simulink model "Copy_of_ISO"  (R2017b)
settings: Solver=FixedStepDiscrete  StartTime=0.0  StopTime=10.0  FixedStep=0.01  RelTol=1e-3  EnableMultiTasking=on
undefined symbols (not defined in the file): ASWTYPE_FALSE, ASWTYPE_TRUE, CcISO_CTCOnlineDelayTime_ms, CcISO_FirLvlDebTime_ms, CcISO_FirLvlResChrg_kohm, CcISO_FirLvlResNotChrg_kohm, CcISO_InitDiagDebMaxTi_ms, CcISO_InitDiagDebTi_ms, CcISO_IsoDefaultValue_kohm, CcISO_IsoMeasDelayTime_ms, CcISO_ISONegVoltDebTime_ms, CcISO_ISONegVoltFliterDiff_V, CcISO_ISOPackVoltMax_V, CcISO_ISOPackVoltMin_V, CcISO_ISOResCnfFltCnt_NUMB, CcISO_ISOResCnfFltVal_kohm, CcISO_ISOResCnfWarnCnt_NUMB, CcISO_ISOResCnfWarnVal_kohm, CcISO_ISOResNvmMin_kohm, CcISO_IsoResVldVal_NUMB, CcISO_ISOSlopeDelayTime_ms, CcISO_ISOSlopeFilterVal_NUMB, CcISO_NegStMeasFiltTi_ms, CcISO_NegVoltHighRat_pct, CcISO_NegVoltLowRat_pct, CcISO_NorLvlResChrg_kohm, CcISO_NorLvlResNotChrg_kohm, CcISO_PosStMeasFiltTi_ms, CcISO_SedLvlDebTime_ms, CcISO_SedLvlResChrg_kohm, CcISO_SedLvlResNotChrg_kohm, Enum_CTCCtrCtlConnMode, Enum_CTCCtrCtlState, Enum_ISOHVIsoFltLevel, Enum_ISOHVIsoMeasState, Enum_LDPCC2St, Enum_MSMBMUState, ISO_CONST0_NUMB, ISO_CONST1000_NUMB, ISO_CONST1_NUMB, ISO_RESRB1_OHM, ISO_RESRB2_OHM, ISO_RESRS1_OHM, ISO_RESRS2_OHM, ISO_RUNTIME_MS
libraries: AIWAYS_Powertrain_BMS_lib x48
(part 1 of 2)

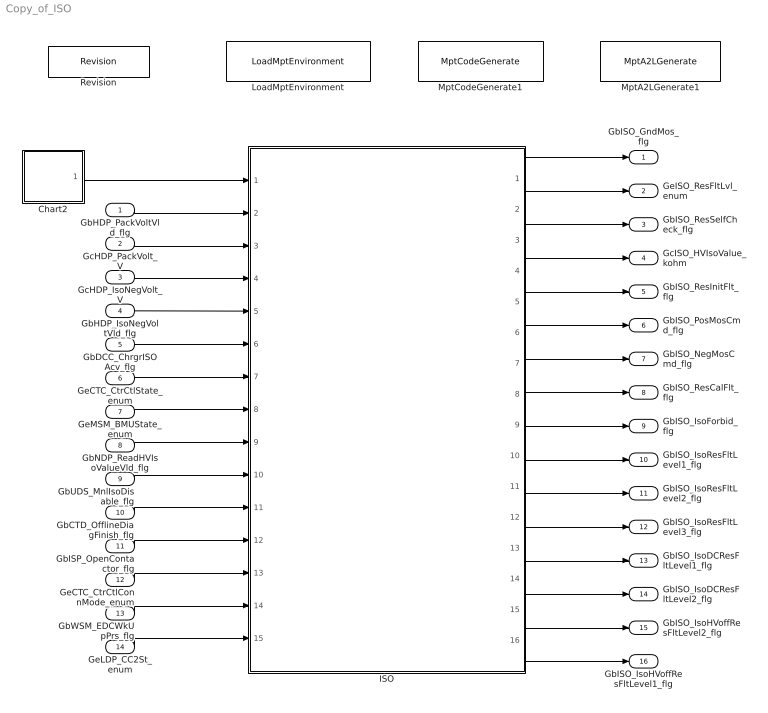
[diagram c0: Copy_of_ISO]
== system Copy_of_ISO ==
  GbHDP_PackVoltVld_flg : Inport
  GcHDP_PackVolt_V : Inport  Port=2
  GcHDP_IsoNegVolt_V : Inport  Port=3
  GbHDP_IsoNegVoltVld_flg : Inport  Port=4
  GbDCC_ChrgrISOAcv_flg : Inport  Port=5
  GeCTC_CtrCtlState_enum : Inport  Port=6
  GeMSM_BMUState_enum : Inport  Port=7
  GbNDP_ReadHVIsoValueVld_flg : Inport  Port=8
  GbUDS_MnlIsoDisable_flg : Inport  Port=9
  GbCTD_OfflineDiagFinish_flg : Inport  Port=10
  GbISP_OpenContactor_flg : Inport  Port=11
  GeCTC_CtrCtlConnMode_enum : Inport  Port=12
  GbWSM_EDCWkUpPrs_flg : Inport  Port=13
  GeLDP_CC2St_enum : Inport  Port=14
  Chart2 : Stateflow chart  TreatAsAtomicUnit=on
  ISO : Subsystem
  LoadMptEnvironment : AIWAYS_Powertrain_BMS_lib/Config/LoadMptEnvironment  ProjectName=Comm  SuppierID=NewPlatformUAES
  MptA2LGenerate1 : AIWAYS_Powertrain_BMS_lib/Config/MptA2LGenerate  SystemSampleTime=-1
  MptCodeGenerate1 : AIWAYS_Powertrain_BMS_lib/Config/MptCodeGenerate  SystemSampleTime=-1
  Revision : AIWAYS_Powertrain_BMS_lib/Config/Revision  curVersion='M110C108R107'  newVersion='M110C108R107'
  GbISO_GndMos_flg : Outport
  GeISO_ResFltLvl_enum : Outport  Port=2
  GbISO_ResSelfCheck_flg : Outport  Port=3
  GcISO_HVIsoValue_kohm : Outport  Port=4
  GbISO_ResInitFlt_flg : Outport  Port=5
  GbISO_PosMosCmd_flg : Outport  Port=6
  GbISO_NegMosCmd_flg : Outport  Port=7
  GbISO_ResCalFlt_flg : Outport  Port=8
  GbISO_IsoForbid_flg : Outport  Port=9
  GbISO_IsoResFltLevel1_flg : Outport  Port=10
  GbISO_IsoResFltLevel2_flg : Outport  Port=11
  GbISO_IsoResFltLevel3_flg : Outport  Port=12
  GbISO_IsoDCResFltLevel1_flg : Outport  Port=13
  GbISO_IsoDCResFltLevel2_flg : Outport  Port=14
  GbISO_IsoHVoffResFltLevel2_flg : Outport  Port=15
  GbISO_IsoHVoffResFltLevel1_flg : Outport  Port=16
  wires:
  Chart2/1(ISO_Insulation_100ms()) -> ISO/1(ISO_Insulation_100ms)
  GbHDP_PackVoltVld_flg/1 -> ISO/2(GbHDP_PackVoltVld_flg)
  GcHDP_PackVolt_V/1 -> ISO/3(GcHDP_PackVolt_V)
  GcHDP_IsoNegVolt_V/1 -> ISO/4(GcHDP_IsoNegVolt_V)
  GbHDP_IsoNegVoltVld_flg/1 -> ISO/5(GbHDP_IsoNegVoltVld_flg)
  GbDCC_ChrgrISOAcv_flg/1 -> ISO/6(GbDCC_ChrgrISOAcv_flg)
  GeCTC_CtrCtlState_enum/1 -> ISO/7(GeCTC_CtrCtlState_enum)
  GeMSM_BMUState_enum/1 -> ISO/8(GeMSM_BMUState_enum)
  GbNDP_ReadHVIsoValueVld_flg/1 -> ISO/9(GbNDP_ReadHVIsoValueVld_flg)
  GbUDS_MnlIsoDisable_flg/1 -> ISO/10(GbUDS_MnlIsoDisable_flg)
  GbCTD_OfflineDiagFinish_flg/1 -> ISO/11(GbCTD_OfflineDiagFinish_flg)
  GbISP_OpenContactor_flg/1 -> ISO/12(GbISP_OpenContactor_flg)
  GeCTC_CtrCtlConnMode_enum/1 -> ISO/13(GeCTC_CtrCtlConnMode_enum)
  ISO/1(GbISO_GndMos_flg) -> GbISO_GndMos_flg/1
  ISO/2(GeISO_ResFltLvl_enum) -> GeISO_ResFltLvl_enum/1
  ISO/3(GbISO_ResSelfCheck_flg) -> GbISO_ResSelfCheck_flg/1
  ISO/4(GcISO_HVIsoValue_kohm) -> GcISO_HVIsoValue_kohm/1
  ISO/5(GbISO_ResInitFlt_flg) -> GbISO_ResInitFlt_flg/1
  ISO/6(GbISO_PosMosCmd_flg) -> GbISO_PosMosCmd_flg/1
  ISO/7(GbISO_NegMosCmd_flg) -> GbISO_NegMosCmd_flg/1
  ISO/8(GbISO_ResCalFlt_flg) -> GbISO_ResCalFlt_flg/1
  GbWSM_EDCWkUpPrs_flg/1 -> ISO/14(GbWSM_EDCWkUpPrs_flg)
  ISO/9(GbISO_IsoForbid_flg) -> GbISO_IsoForbid_flg/1
  ISO/10(GbISO_IsoResFltLevel1_flg) -> GbISO_IsoResFltLevel1_flg/1
  ISO/11(GbISO_IsoResFltLevel2_flg) -> GbISO_IsoResFltLevel2_flg/1
  ISO/12(GbISO_IsoResFltLevel3_flg) -> GbISO_IsoResFltLevel3_flg/1
  GeLDP_CC2St_enum/1 -> ISO/15(GeLDP_CC2St_enum)
  ISO/13(GbISO_IsoDCResFltLevel1_flg) -> GbISO_IsoDCResFltLevel1_flg/1
  ISO/14(GbISO_IsoDCResFltLevel2_flg) -> GbISO_IsoDCResFltLevel2_flg/1
  ISO/15(GbISO_IsoHVoffResFltLevel2_flg) -> GbISO_IsoHVoffResFltLevel2_flg/1
  ISO/16(GbISO_IsoHVoffResFltLevel1_flg) -> GbISO_IsoHVoffResFltLevel1_flg/1

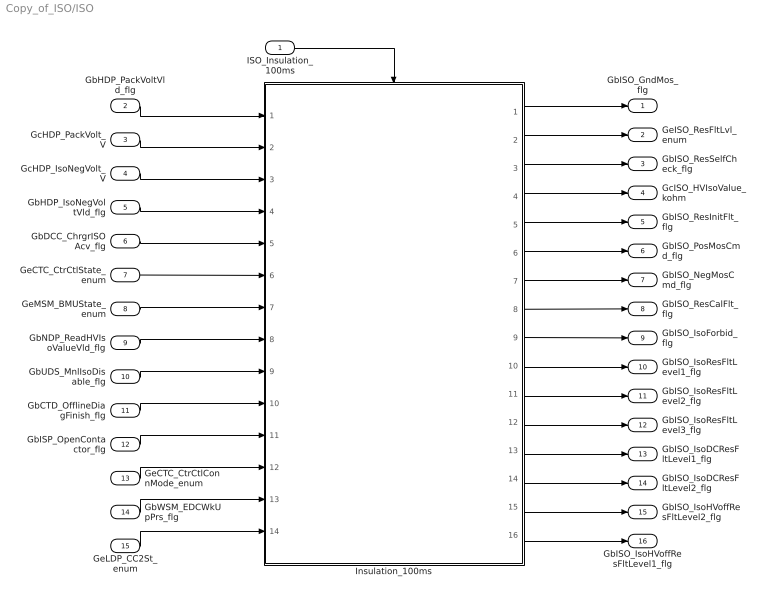
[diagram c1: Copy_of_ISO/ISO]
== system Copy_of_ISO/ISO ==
  ISO_Insulation_100ms : Inport
  GbHDP_PackVoltVld_flg : Inport  Port=2
  GcHDP_PackVolt_V : Inport  Port=3
  GcHDP_IsoNegVolt_V : Inport  Port=4
  GbHDP_IsoNegVoltVld_flg : Inport  Port=5
  GbDCC_ChrgrISOAcv_flg : Inport  Port=6
  GeCTC_CtrCtlState_enum : Inport  Port=7
  GeMSM_BMUState_enum : Inport  Port=8
  GbNDP_ReadHVIsoValueVld_flg : Inport  Port=9
  GbUDS_MnlIsoDisable_flg : Inport  Port=10
  GbCTD_OfflineDiagFinish_flg : Inport  Port=11
  GbISP_OpenContactor_flg : Inport  Port=12
  GeCTC_CtrCtlConnMode_enum : Inport  Port=13
  GbWSM_EDCWkUpPrs_flg : Inport  Port=14
  GeLDP_CC2St_enum : Inport  Port=15
  Insulation_100ms : Subsystem
  GbISO_GndMos_flg : Outport
  GeISO_ResFltLvl_enum : Outport  Port=2
  GbISO_ResSelfCheck_flg : Outport  Port=3
  GcISO_HVIsoValue_kohm : Outport  Port=4
  GbISO_ResInitFlt_flg : Outport  Port=5
  GbISO_PosMosCmd_flg : Outport  Port=6
  GbISO_NegMosCmd_flg : Outport  Port=7
  GbISO_ResCalFlt_flg : Outport  Port=8
  GbISO_IsoForbid_flg : Outport  Port=9
  GbISO_IsoResFltLevel1_flg : Outport  Port=10
  GbISO_IsoResFltLevel2_flg : Outport  Port=11
  GbISO_IsoResFltLevel3_flg : Outport  Port=12
  GbISO_IsoDCResFltLevel1_flg : Outport  Port=13
  GbISO_IsoDCResFltLevel2_flg : Outport  Port=14
  GbISO_IsoHVoffResFltLevel2_flg : Outport  Port=15
  GbISO_IsoHVoffResFltLevel1_flg : Outport  Port=16
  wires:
  ISO_Insulation_100ms/1 -> Insulation_100ms/Trigger
  Insulation_100ms/1(GbISO_GndMos_flg) -> GbISO_GndMos_flg/1
  Insulation_100ms/2(GeISO_ResFltLvl_enum) -> GeISO_ResFltLvl_enum/1
  Insulation_100ms/3(GbISO_ResSelfCheck_flg) -> GbISO_ResSelfCheck_flg/1
  Insulation_100ms/4(GcISO_HVIsoValue_kohm) -> GcISO_HVIsoValue_kohm/1
  Insulation_100ms/5(GbISO_ResInitFlt_flg) -> GbISO_ResInitFlt_flg/1
  Insulation_100ms/6(GbISO_PosMosCmd_flg) -> GbISO_PosMosCmd_flg/1
  Insulation_100ms/7(GbISO_NegMosCmd_flg) -> GbISO_NegMosCmd_flg/1
  Insulation_100ms/8(GbISO_ResCalFlt_flg) -> GbISO_ResCalFlt_flg/1
  GbHDP_PackVoltVld_flg/1 -> Insulation_100ms/1(GbHDP_PackVoltVld_flg)
  GcHDP_PackVolt_V/1 -> Insulation_100ms/2(GcHDP_PackVolt_V)
  GcHDP_IsoNegVolt_V/1 -> Insulation_100ms/3(GcHDP_IsoNegVolt_V)
  GbHDP_IsoNegVoltVld_flg/1 -> Insulation_100ms/4(GbHDP_IsoNegVoltVld_flg)
  GbDCC_ChrgrISOAcv_flg/1 -> Insulation_100ms/5(GbDCC_ChrgrISOAcv_flg)
  GeCTC_CtrCtlState_enum/1 -> Insulation_100ms/6(GeCTC_CtrCtlState_enum)
  GeMSM_BMUState_enum/1 -> Insulation_100ms/7(GeMSM_BMUState_enum)
  GbNDP_ReadHVIsoValueVld_flg/1 -> Insulation_100ms/8(GbNDP_ReadHVIsoValueVld_flg)
  GbUDS_MnlIsoDisable_flg/1 -> Insulation_100ms/9(GbUDS_MnlIsoDisable_flg)
  GbCTD_OfflineDiagFinish_flg/1 -> Insulation_100ms/10(GbCTD_OfflineDiagFinish_flg)
  GbISP_OpenContactor_flg/1 -> Insulation_100ms/11(GbISP_OpenContactor_flg)
  GeCTC_CtrCtlConnMode_enum/1 -> Insulation_100ms/12(GeCTC_CtrCtlConnMode_enum)
  GbWSM_EDCWkUpPrs_flg/1 -> Insulation_100ms/13(GbWSM_EDCWkUpPrs_flg)
  Insulation_100ms/9(GbISO_IsoForbid_flg) -> GbISO_IsoForbid_flg/1
  Insulation_100ms/10(GbISO_IsoResFltLevel1_flg) -> GbISO_IsoResFltLevel1_flg/1
  Insulation_100ms/11(GbISO_IsoResFltLevel2_flg) -> GbISO_IsoResFltLevel2_flg/1
  Insulation_100ms/12(GbISO_IsoResFltLevel3_flg) -> GbISO_IsoResFltLevel3_flg/1
  GeLDP_CC2St_enum/1 -> Insulation_100ms/14(GeLDP_CC2St_enum)
  Insulation_100ms/13(GbISO_IsoDCResFltLevel1_flg) -> GbISO_IsoDCResFltLevel1_flg/1
  Insulation_100ms/14(GbISO_IsoDCResFltLevel2_flg) -> GbISO_IsoDCResFltLevel2_flg/1
  Insulation_100ms/15(GbISO_IsoHVoffResFltLevel2_flg) -> GbISO_IsoHVoffResFltLevel2_flg/1
  Insulation_100ms/16(GbISO_IsoHVoffResFltLevel1_flg) -> GbISO_IsoHVoffResFltLevel1_flg/1

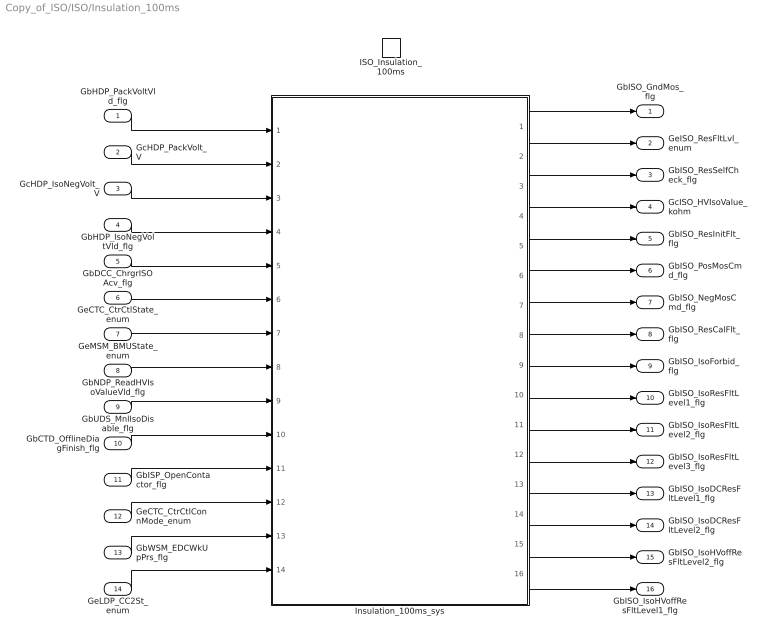
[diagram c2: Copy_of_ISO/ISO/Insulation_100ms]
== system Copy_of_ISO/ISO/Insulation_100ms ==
  GbHDP_PackVoltVld_flg : Inport
  GcHDP_PackVolt_V : Inport  Port=2
  GcHDP_IsoNegVolt_V : Inport  Port=3
  GbHDP_IsoNegVoltVld_flg : Inport  Port=4
  GbDCC_ChrgrISOAcv_flg : Inport  Port=5
  GeCTC_CtrCtlState_enum : Inport  Port=6
  GeMSM_BMUState_enum : Inport  Port=7
  GbNDP_ReadHVIsoValueVld_flg : Inport  Port=8
  GbUDS_MnlIsoDisable_flg : Inport  Port=9
  GbCTD_OfflineDiagFinish_flg : Inport  Port=10
  GbISP_OpenContactor_flg : Inport  Port=11
  GeCTC_CtrCtlConnMode_enum : Inport  Port=12
  GbWSM_EDCWkUpPrs_flg : Inport  Port=13
  GeLDP_CC2St_enum : Inport  Port=14
  ISO_Insulation_100ms : TriggerPort  TriggerType=function-call  VariantControl=(inherit)
  Insulation_100ms_sys : Subsystem
  GbISO_GndMos_flg : Outport
  GeISO_ResFltLvl_enum : Outport  Port=2
  GbISO_ResSelfCheck_flg : Outport  Port=3
  GcISO_HVIsoValue_kohm : Outport  Port=4
  GbISO_ResInitFlt_flg : Outport  Port=5
  GbISO_PosMosCmd_flg : Outport  Port=6
  GbISO_NegMosCmd_flg : Outport  Port=7
  GbISO_ResCalFlt_flg : Outport  Port=8
  GbISO_IsoForbid_flg : Outport  Port=9
  GbISO_IsoResFltLevel1_flg : Outport  Port=10
  GbISO_IsoResFltLevel2_flg : Outport  Port=11
  GbISO_IsoResFltLevel3_flg : Outport  Port=12
  GbISO_IsoDCResFltLevel1_flg : Outport  Port=13
  GbISO_IsoDCResFltLevel2_flg : Outport  Port=14
  GbISO_IsoHVoffResFltLevel2_flg : Outport  Port=15
  GbISO_IsoHVoffResFltLevel1_flg : Outport  Port=16
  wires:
  Insulation_100ms_sys/1(GbISO_GndMos_flg) -> GbISO_GndMos_flg/1
  Insulation_100ms_sys/2(GeISO_ResFltLvl_enum) -> GeISO_ResFltLvl_enum/1
  Insulation_100ms_sys/3(GbISO_ResSelfCheck_flg) -> GbISO_ResSelfCheck_flg/1
  Insulation_100ms_sys/4(GcISO_HVIsoValue_kohm) -> GcISO_HVIsoValue_kohm/1
  Insulation_100ms_sys/5(GbISO_ResInitFlt_flg) -> GbISO_ResInitFlt_flg/1
  Insulation_100ms_sys/6(GbISO_PosMosCmd_flg) -> GbISO_PosMosCmd_flg/1
  Insulation_100ms_sys/7(GbISO_NegMosCmd_flg) -> GbISO_NegMosCmd_flg/1
  Insulation_100ms_sys/8(GbISO_ResCalFlt_flg) -> GbISO_ResCalFlt_flg/1
  GbHDP_PackVoltVld_flg/1 -> Insulation_100ms_sys/1(GbHDP_PackVoltVld_flg)
  GcHDP_PackVolt_V/1 -> Insulation_100ms_sys/2(GcHDP_PackVolt_V)
  GcHDP_IsoNegVolt_V/1 -> Insulation_100ms_sys/3(GcHDP_IsoNegVolt_V)
  GbHDP_IsoNegVoltVld_flg/1 -> Insulation_100ms_sys/4(GbHDP_IsoNegVoltVld_flg)
  GbDCC_ChrgrISOAcv_flg/1 -> Insulation_100ms_sys/5(GbDCC_ChrgrISOAcv_flg)
  GeCTC_CtrCtlState_enum/1 -> Insulation_100ms_sys/6(GeCTC_CtrCtlState_enum)
  GeMSM_BMUState_enum/1 -> Insulation_100ms_sys/7(GeMSM_BMUState_enum)
  GbNDP_ReadHVIsoValueVld_flg/1 -> Insulation_100ms_sys/8(GbNDP_ReadHVIsoValueVld_flg)
  GbUDS_MnlIsoDisable_flg/1 -> Insulation_100ms_sys/9(GbUDS_MnlIsoDisable_flg)
  GbCTD_OfflineDiagFinish_flg/1 -> Insulation_100ms_sys/10(GbCTD_OfflineDiagFinish_flg)
  GbISP_OpenContactor_flg/1 -> Insulation_100ms_sys/11(GbISP_OpenContactor_flg)
  GeCTC_CtrCtlConnMode_enum/1 -> Insulation_100ms_sys/12(GeCTC_CtrCtlConnMode_enum)
  GbWSM_EDCWkUpPrs_flg/1 -> Insulation_100ms_sys/13(GbWSM_EDCWkUpPrs_flg)
  Insulation_100ms_sys/9(GbISO_IsoForbid_flg) -> GbISO_IsoForbid_flg/1
  Insulation_100ms_sys/10(GbISO_IsoResFltLevel1_flg) -> GbISO_IsoResFltLevel1_flg/1
  Insulation_100ms_sys/11(GbISO_IsoResFltLevel2_flg) -> GbISO_IsoResFltLevel2_flg/1
  Insulation_100ms_sys/12(GbISO_IsoResFltLevel3_flg) -> GbISO_IsoResFltLevel3_flg/1
  GeLDP_CC2St_enum/1 -> Insulation_100ms_sys/14(GeLDP_CC2St_enum)
  Insulation_100ms_sys/13(GbISO_IsoDCResFltLevel1_flg) -> GbISO_IsoDCResFltLevel1_flg/1
  Insulation_100ms_sys/14(GbISO_IsoDCResFltLevel2_flg) -> GbISO_IsoDCResFltLevel2_flg/1
  Insulation_100ms_sys/15(GbISO_IsoHVoffResFltLevel2_flg) -> GbISO_IsoHVoffResFltLevel2_flg/1
  Insulation_100ms_sys/16(GbISO_IsoHVoffResFltLevel1_flg) -> GbISO_IsoHVoffResFltLevel1_flg/1

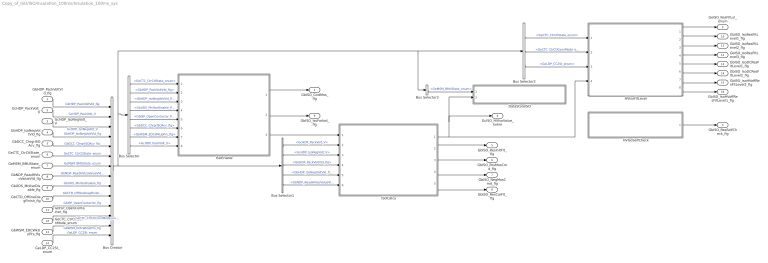
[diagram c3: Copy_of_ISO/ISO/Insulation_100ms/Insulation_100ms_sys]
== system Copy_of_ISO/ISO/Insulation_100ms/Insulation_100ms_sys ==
  GbHDP_PackVoltVld_flg : Inport
  GcHDP_PackVolt_V : Inport  Port=2
  GcHDP_IsoNegVolt_V : Inport  Port=3
  GbHDP_IsoNegVoltVld_flg : Inport  Port=4
  GbDCC_ChrgrISOAcv_flg : Inport  Port=5
  GeCTC_CtrCtlState_enum : Inport  Port=6
  GeMSM_BMUState_enum : Inport  Port=7
  GbNDP_ReadHVIsoValueVld_flg : Inport  Port=8
  GbUDS_MnlIsoDisable_flg : Inport  Port=9
  GbCTD_OfflineDiagFinish_flg : Inport  Port=10
  GbISP_OpenContactor_flg : Inport  Port=11
  GeCTC_CtrCtlConnMode_enum : Inport  Port=12
  GbWSM_EDCWkUpPrs_flg : Inport  Port=13
  GeLDP_CC2St_enum : Inport  Port=14
  Bus Creator : BusCreator  Inputs=14
  Bus Selector : BusSelector  OutputSignals=GeCTC_CtrCtlState_enum,GbHDP_PackVoltVld_flg,GbHDP_IsoNegVoltVld_flg,GbUDS_MnlIsoDisable_flg,GbISP_OpenContactor_flg,GbDCC_ChrgrISOAcv_flg,GbWSM_EDCWkUpPrs_flg,GcHDP_PackVolt_V
  Bus Selector1 : BusSelector  OutputSignals=GcHDP_PackVolt_V,GcHDP_IsoNegVolt_V,GbHDP_PackVoltVld_flg,GbHDP_IsoNegVoltVld_flg,GbNDP_ReadHVIsoValueVld_flg
  Bus Selector2 : BusSelector  OutputSignals=GeCTC_CtrCtlState_enum,GeCTC_CtrCtlConnMode_enum,GeLDP_CC2St_enum
  Bus Selector3 : BusSelector  OutputSignals=GeMSM_BMUState_enum
  DataStoreISO : Subsystem
  HVIsoFltLevel : Subsystem
  HVIsoSelfCheck : Subsystem
  ISOCalcu : Subsystem
  ISOEnable : Subsystem
  GbISO_GndMos_flg : Outport
  GeISO_ResFltLvl_enum : Outport  Port=2
  GbISO_ResSelfCheck_flg : Outport  Port=3
  GcISO_HVIsoValue_kohm : Outport  Port=4
  GbISO_ResInitFlt_flg : Outport  Port=5
  GbISO_PosMosCmd_flg : Outport  Port=6
  GbISO_NegMosCmd_flg : Outport  Port=7
  GbISO_ResCalFlt_flg : Outport  Port=8
  GbISO_IsoForbid_flg : Outport  Port=9
  GbISO_IsoResFltLevel1_flg : Outport  Port=10
  GbISO_IsoResFltLevel2_flg : Outport  Port=11
  GbISO_IsoResFltLevel3_flg : Outport  Port=12
  GbISO_IsoDCResFltLevel1_flg : Outport  Port=13
  GbISO_IsoDCResFltLevel2_flg : Outport  Port=14
  GbISO_IsoHVoffResFltLevel2_flg : Outport  Port=15
  GbISO_IsoHVoffResFltLevel1_flg : Outport  Port=16
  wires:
  GbHDP_PackVoltVld_flg/1 -> Bus Creator/1  "GbHDP_PackVoltVld_flg"
  GcHDP_PackVolt_V/1 -> Bus Creator/2  "GcHDP_PackVolt_V"
  GcHDP_IsoNegVolt_V/1 -> Bus Creator/3  "GcHDP_IsoNegVolt_V"
  GbHDP_IsoNegVoltVld_flg/1 -> Bus Creator/4  "GbHDP_IsoNegVoltVld_flg"
  GbDCC_ChrgrISOAcv_flg/1 -> Bus Creator/5  "GbDCC_ChrgrISOAcv_flg"
  GeCTC_CtrCtlState_enum/1 -> Bus Creator/6  "GeCTC_CtrCtlState_enum"
  GeMSM_BMUState_enum/1 -> Bus Creator/7  "GeMSM_BMUState_enum"
  GbNDP_ReadHVIsoValueVld_flg/1 -> Bus Creator/8  "GbNDP_ReadHVIsoValueVld_flg"
  GbUDS_MnlIsoDisable_flg/1 -> Bus Creator/9  "GbUDS_MnlIsoDisable_flg"
  GbCTD_OfflineDiagFinish_flg/1 -> Bus Creator/10  "GbCTD_OfflineDiagFinish_flg"
  Bus Selector/1 -> ISOEnable/1(GeCTC_CtrCtlState_enum)  "<GeCTC_CtrCtlState_enum>"
  Bus Selector/2 -> ISOEnable/2(GbHDP_PackVoltVld_flg)  "<GbHDP_PackVoltVld_flg>"
  Bus Selector/3 -> ISOEnable/3(GbHDP_IsoNegVoltVld_flg)  "<GbHDP_IsoNegVoltVld_flg>"
  Bus Selector/4 -> ISOEnable/4(GbUDS_MnlIsoDisable_flg)  "<GbUDS_MnlIsoDisable_flg>"
  Bus Selector/5 -> ISOEnable/5(GbISP_OpenContactor_flg)  "<GbISP_OpenContactor_flg>"
  Bus Selector/6 -> ISOEnable/6(GbDCC_ChrgrISOAcv_flg)  "<GbDCC_ChrgrISOAcv_flg>"
  ISOEnable/3(LbISO_IsoForbid_flg) -> ISOCalcu/1(LbISO_IsoForbid_flg)
  Bus Selector1/1 -> ISOCalcu/2(GcHDP_PackVolt_V)  "<GcHDP_PackVolt_V>"
  Bus Selector1/2 -> ISOCalcu/3(GcHDP_IsoNegVolt_V)  "<GcHDP_IsoNegVolt_V>"
  Bus Selector1/3 -> ISOCalcu/4(GbHDP_PackVoltVld_flg)  "<GbHDP_PackVoltVld_flg>"
  Bus Selector1/4 -> ISOCalcu/5(GbHDP_IsoNegVoltVld_flg)  "<GbHDP_IsoNegVoltVld_flg>"
  ISOEnable/1(GbISO_GndMos_flg) -> GbISO_GndMos_flg/1
  Bus Selector1/5 -> ISOCalcu/6(GbNDP_ReadHVIsoValueVld_flg)  "<GbNDP_ReadHVIsoValueVld_flg>"
  ISOCalcu/1(GcISO_HVIsoValue_kohm) -> GcISO_HVIsoValue_kohm/1, DataStoreISO/2(GcISO_HVIsoValue_kohm), HVIsoFltLevel/4(GcISO_HVIsoValue_kohm)
  GeCTC_CtrCtlConnMode_enum/1 -> Bus Creator/12  "GeCTC_CtrCtlConnMode_enum"
  Bus Selector2/1 -> HVIsoFltLevel/1(GeCTC_CtrCtlState_enum)  "<GeCTC_CtrCtlState_enum>"
  Bus Selector2/2 -> HVIsoFltLevel/2(GeCTC_CtrCtlConnMode_enum)  "<GeCTC_CtrCtlConnMode_enum>"
  Bus Creator/1 -> Bus Selector3/1, Bus Selector2/1, Bus Selector/1, Bus Selector1/1
  Bus Selector3/1 -> DataStoreISO/1(GeMSM_BMUState_enum)  "<GeMSM_BMUState_enum>"
  HVIsoFltLevel/1(GeISO_ResFltLvl_enum) -> GeISO_ResFltLvl_enum/1
  HVIsoSelfCheck/1(GbISO_ResSelfCheck_flg) -> GbISO_ResSelfCheck_flg/1
  ISOCalcu/2(GbISO_ResInitFlt_flg) -> GbISO_ResInitFlt_flg/1
  ISOCalcu/3(GbISO_PosMosCmd_flg) -> GbISO_PosMosCmd_flg/1
  ISOCalcu/4(GbISO_NegMosCmd_flg) -> GbISO_NegMosCmd_flg/1
  ISOCalcu/5(GbISO_ResCalFlt_flg) -> GbISO_ResCalFlt_flg/1
  GbWSM_EDCWkUpPrs_flg/1 -> Bus Creator/13  "GbWSM_EDCWkUpPrs_flg"
  Bus Selector/7 -> ISOEnable/7(GbWSM_EDCWkUpPrs_flg)  "<GbWSM_EDCWkUpPrs_flg>"
  ISOEnable/2(GbISO_IsoForbid_flg) -> GbISO_IsoForbid_flg/1
  HVIsoFltLevel/2(GbISO_IsoResFltLevel1_flg) -> GbISO_IsoResFltLevel1_flg/1
  HVIsoFltLevel/3(GbISO_IsoResFltLevel2_flg) -> GbISO_IsoResFltLevel2_flg/1
  HVIsoFltLevel/4(GbISO_IsoResFltLevel3_flg) -> GbISO_IsoResFltLevel3_flg/1
  Bus Selector/8 -> ISOEnable/8(GcHDP_PackVolt_V)  "<GcHDP_PackVolt_V>"
  GbISP_OpenContactor_flg/1 -> Bus Creator/11  "GbISP_OpenContactor_flg"
  GeLDP_CC2St_enum/1 -> Bus Creator/14  "GeLDP_CC2St_enum"
  Bus Selector2/3 -> HVIsoFltLevel/3(GeLDP_CC2St_enum)  "<GeLDP_CC2St_enum>"
  HVIsoFltLevel/5(GbISO_IsoDCResFltLevel1_flg) -> GbISO_IsoDCResFltLevel1_flg/1
  HVIsoFltLevel/6(GbISO_IsoDCResFltLevel2_flg) -> GbISO_IsoDCResFltLevel2_flg/1
  HVIsoFltLevel/7(GbISO_IsoHVoffResFltLevel2_flg) -> GbISO_IsoHVoffResFltLevel2_flg/1
  HVIsoFltLevel/8(GbISO_IsoHVoffResFltLevel1_flg) -> GbISO_IsoHVoffResFltLevel1_flg/1

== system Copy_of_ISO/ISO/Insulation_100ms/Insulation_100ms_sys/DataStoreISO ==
  GeMSM_BMUState_enum : Inport
  GcISO_HVIsoValue_kohm : Inport  Port=2
  Constant3 : Constant  Value=Enum_MSMBMUState.Enum_MSMBMUState_Shutdown
  Data Type Conversion1 : DataTypeConversion
  DataStoreISO_Work : Subsystem
  Relational Operator3 : RelationalOperator  Operator===  OutDataTypeStr=boolean
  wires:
  GcISO_HVIsoValue_kohm/1 -> DataStoreISO_Work/1(GcISO_HVIsoValue_kohm)
  GeMSM_BMUState_enum/1 -> Data Type Conversion1/1
  Relational Operator3/1 -> DataStoreISO_Work/Enable  "LbISO_DataStoreEN_flg"
  Constant3/1 -> Relational Operator3/2
  Data Type Conversion1/1 -> Relational Operator3/1

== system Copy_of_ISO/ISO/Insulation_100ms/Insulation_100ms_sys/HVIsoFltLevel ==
  GeCTC_CtrCtlState_enum : Inport
  GeCTC_CtrCtlConnMode_enum : Inport  Port=2
  GeLDP_CC2St_enum : Inport  Port=3
  GcISO_HVIsoValue_kohm : Inport  Port=4
  ISOFlt : Subsystem
  IsoLevelResThrld : Subsystem
  GeISO_ResFltLvl_enum : Outport
  GbISO_IsoResFltLevel1_flg : Outport  Port=2
  GbISO_IsoResFltLevel2_flg : Outport  Port=3
  GbISO_IsoResFltLevel3_flg : Outport  Port=4
  GbISO_IsoDCResFltLevel1_flg : Outport  Port=5
  GbISO_IsoDCResFltLevel2_flg : Outport  Port=6
  GbISO_IsoHVoffResFltLevel2_flg : Outport  Port=7
  GbISO_IsoHVoffResFltLevel1_flg : Outport  Port=8
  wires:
  GcISO_HVIsoValue_kohm/1 -> ISOFlt/1(GcISO_HVIsoValue_kohm)
  GeCTC_CtrCtlState_enum/1 -> IsoLevelResThrld/1(GeCTC_CtrCtlState_enum), ISOFlt/3(GeCTC_CtrCtlState_enum)
  IsoLevelResThrld/1(LcISO_IsoSecondLevelResThrld_kohm) -> ISOFlt/4(LcISO_IsoSecondLevelResThrld_kohm)
  IsoLevelResThrld/2(LcISO_IsoFirstLevelResThrld_kohm) -> ISOFlt/5(LcISO_IsoFirstLevelResThrld_kohm)
  IsoLevelResThrld/3(LcISO_IsoNormalLevelResThrld_kohm) -> ISOFlt/6(LcISO_IsoNormalLevelResThrld_kohm)
  GeCTC_CtrCtlConnMode_enum/1 -> IsoLevelResThrld/2(GeCTC_CtrCtlConnMode_enum)
  ISOFlt/1(GeISO_ResFltLvl_enum) -> GeISO_ResFltLvl_enum/1
  ISOFlt/2(GbISO_IsoResFltLevel1_flg) -> GbISO_IsoResFltLevel1_flg/1
  ISOFlt/3(GbISO_IsoResFltLevel2_flg) -> GbISO_IsoResFltLevel2_flg/1
  ISOFlt/4(GbISO_IsoResFltLevel3_flg) -> GbISO_IsoResFltLevel3_flg/1
  GeLDP_CC2St_enum/1 -> ISOFlt/2(GeLDP_CC2St_enum)
  ISOFlt/5(GbISO_IsoDCResFltLevel1_flg) -> GbISO_IsoDCResFltLevel1_flg/1
  ISOFlt/6(GbISO_IsoDCResFltLevel2_flg) -> GbISO_IsoDCResFltLevel2_flg/1
  ISOFlt/7(GbISO_IsoHVoffResFltLevel2_flg) -> GbISO_IsoHVoffResFltLevel2_flg/1
  ISOFlt/8(GbISO_IsoHVoffResFltLevel1_flg) -> GbISO_IsoHVoffResFltLevel1_flg/1

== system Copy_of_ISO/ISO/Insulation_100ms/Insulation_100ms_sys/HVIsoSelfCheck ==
  Constant7 : Constant  Value=ASWTYPE_TRUE
  ISO_GbISO_ResSelfCheck_flg : AIWAYS_Powertrain_BMS_lib/Signals/OverWrite  OverWrite_Value=CbISO_ResSelfCheckOvr_flg  OverWrite_flag=CbISO_ResSelfCheckOvrSwt_flg
  GbISO_ResSelfCheck_flg : Outport
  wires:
  Constant7/1 -> ISO_GbISO_ResSelfCheck_flg/1
  ISO_GbISO_ResSelfCheck_flg/1 -> GbISO_ResSelfCheck_flg/1  "GbISO_ResSelfCheck_flg"

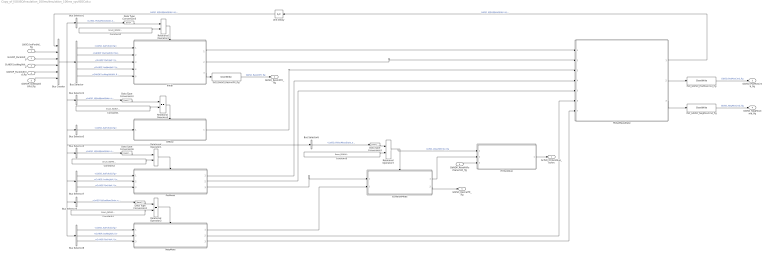
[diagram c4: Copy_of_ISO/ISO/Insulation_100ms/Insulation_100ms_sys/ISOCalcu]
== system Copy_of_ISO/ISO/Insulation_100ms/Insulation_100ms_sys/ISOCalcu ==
  LbISO_IsoForbid_flg : Inport
  GcHDP_PackVolt_V : Inport  Port=2
  GcHDP_IsoNegVolt_V : Inport  Port=3
  GbHDP_PackVoltVld_flg : Inport  Port=4
  GbHDP_IsoNegVoltVld_flg : Inport  Port=5
  GbNDP_ReadHVIsoValueVld_flg : Inport  Port=6
  Bus Creator : BusCreator  Inputs=6
  Bus Selector : BusSelector  OutputSignals=LbISO_IsoForbid_flg,GbHDP_PackVoltVld_flg,GcHDP_PackVolt_V,GcHDP_IsoNegVolt_V,GbHDP_IsoNegVoltVld_flg
  Bus Selector{1..2,4..6} (5 alike) : BusSelector  OutputSignals=LeISO_HVIsoMeasState_enum
  Bus Selector3 : BusSelector  OutputSignals=LbISO_IsoForbid_flg
  Bus Selector7 : BusSelector  OutputSignals=LbISO_IsoForbid_flg,GcHDP_IsoNegVolt_V,GcHDP_PackVolt_V
  Bus Selector8 : BusSelector  OutputSignals=LbISO_IsoForbid_flg,GcHDP_IsoNegVolt_V,GcHDP_PackVolt_V
  Constant1 : Constant  Value=Enum_ISOHVIsoMeasState.Enum_ISOHVIsoMeasState_Offline
  Constant2 : Constant  Value=Enum_ISOHVIsoMeasState.Enum_ISOHVIsoMeasState_PosMeas
  Constant3 : Constant  Value=Enum_ISOHVIsoMeasState.Enum_ISOHVIsoMeasState_NegMeas
  Constant4 : Constant  Value=Enum_ISOHVIsoMeasState.Enum_ISOHVIsoMeasState_Initial
  Constant5 : Constant  Value=Enum_ISOHVIsoMeasState.Enum_ISOHVIsoMeasState_VauleCalcu
  Data Type Conversion{1..3,5..6} (5 alike) : DataTypeConversion
  HVIsoMeasState : Stateflow chart  TreatAsAtomicUnit=on
  HVIsoValue : Subsystem
  ISOValueMeas : Subsystem  TreatAsAtomicUnit=on
  ISO_GbISO_NegMosCmd_flg : AIWAYS_Powertrain_BMS_lib/Signals/OverWrite  OverWrite_Value=CbISO_NegMosCmdOvr_flg  OverWrite_flag=CbISO_NegMosCmdOvrSwt_flg
  ISO_GbISO_PosMosCmd_flg : AIWAYS_Powertrain_BMS_lib/Signals/OverWrite  OverWrite_Value=CbISO_PosMosCmdOvr_flg  OverWrite_flag=CbISO_PosMosCmdOvrSwt_flg
  ISO_GbISO_ResInitFlt_flg : AIWAYS_Powertrain_BMS_lib/Signals/OverWrite  OverWrite_Value=CbISO_ResInitFltOvr_flg  OverWrite_flag=CbISO_ResInitFltOvrSwt_flg
  Initial : Subsystem  TreatAsAtomicUnit=on
  NegMeas : Subsystem  TreatAsAtomicUnit=on
  Offline : Subsystem  TreatAsAtomicUnit=on
  PosMeas : Subsystem  TreatAsAtomicUnit=on
  Relational Operator{1..5} (5 alike) : RelationalOperator  Operator===  OutDataTypeStr=boolean
  Unit Delay : UnitDelay  SampleTime=-1  StateName=StateName
  GcISO_HVIsoValue_kohm : Outport
  GbISO_ResInitFlt_flg : Outport  Port=2
  GbISO_PosMosCmd_flg : Outport  Port=3
  GbISO_NegMosCmd_flg : Outport  Port=4
  GbISO_ResCalFlt_flg : Outport  Port=5
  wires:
  Relational Operator1/1 -> PosMeas/Enable
  Relational Operator2/1 -> NegMeas/Enable
  Constant2/1 -> Relational Operator1/2
  Constant3/1 -> Relational Operator2/2
  HVIsoMeasState/2(GbISO_PosMosCmd_flg) -> ISO_GbISO_PosMosCmd_flg/1
  HVIsoMeasState/3(GbISO_NegMosCmd_flg) -> ISO_GbISO_NegMosCmd_flg/1
  ISOValueMeas/1(LcISO_HVIsoValue_kohm) -> HVIsoValue/2(LcISO_HVIsoValue_kohm)
  HVIsoMeasState/1(LeISO_HVIsoMeasState_enum) -> Unit Delay/1  "LeISO_HVIsoMeasState_enum"
  Data Type Conversion6/1 -> Relational Operator1/1
  Data Type Conversion2/1 -> Relational Operator2/1
  PosMeas/3(LcISO_PosStBeta_numb) -> ISOValueMeas/1(LcISO_PosStBeta_numb)
  NegMeas/1(LcISO_NegStAlpha_numb) -> ISOValueMeas/2(LcISO_NegStAlpha_numb)
  HVIsoValue/1(GcISO_HVIsoValue_kohm) -> GcISO_HVIsoValue_kohm/1
  LbISO_IsoForbid_flg/1 -> Bus Creator/2
  GcHDP_PackVolt_V/1 -> Bus Creator/3
  GcHDP_IsoNegVolt_V/1 -> Bus Creator/4
  GbHDP_PackVoltVld_flg/1 -> Bus Creator/5
  GbHDP_IsoNegVoltVld_flg/1 -> Bus Creator/6
  Unit Delay/1 -> Bus Creator/1  "LeISO_HVIsoMeasState_enum"
  Bus Selector/1 -> Initial/1(LbISO_IsoForbid_flg)  "<LbISO_IsoForbid_flg>"
  Bus Selector/2 -> Initial/2(GbHDP_PackVoltVld_flg)  "<GbHDP_PackVoltVld_flg>"
  Bus Selector/3 -> Initial/3(GcHDP_PackVolt_V)  "<GcHDP_PackVolt_V>"
  Bus Selector/4 -> Initial/4(GcHDP_IsoNegVolt_V)  "<GcHDP_IsoNegVolt_V>"
  Bus Selector/5 -> Initial/5(GbHDP_IsoNegVoltVld_flg)  "<GbHDP_IsoNegVoltVld_flg>"
  Relational Operator4/1 -> Initial/Enable
  Constant4/1 -> Relational Operator4/2
  Data Type Conversion5/1 -> Relational Operator4/1
  Bus Selector1/1 -> Data Type Conversion5/1  "<LeISO_HVIsoMeasState_enum>"
  Bus Selector2/1 -> Data Type Conversion1/1  "<LeISO_HVIsoMeasState_enum>"
  Data Type Conversion1/1 -> Relational Operator5/1
  Constant1/1 -> Relational Operator5/2
  Relational Operator5/1 -> Offline/Enable
  Bus Selector3/1 -> Offline/1(LbISO_IsoForbid_flg)  "<LbISO_IsoForbid_flg>"
  Bus Selector4/1 -> Data Type Conversion6/1  "<LeISO_HVIsoMeasState_enum>"
  Bus Selector5/1 -> Data Type Conversion2/1  "<LeISO_HVIsoMeasState_enum>"
  Bus Selector6/1 -> Data Type Conversion3/1  "<LeISO_HVIsoMeasState_enum>"
  Bus Creator/1 -> Bus Selector8/1, Bus Selector5/1, Bus Selector7/1, Bus Selector4/1, Bus Selector6/1, Bus Selector3/1, Bus Selector2/1, Bus Selector1/1, Bus Selector/1
  Data Type Conversion3/1 -> Relational Operator3/1
  Constant5/1 -> Relational Operator3/2
  Relational Operator3/1 -> HVIsoValue/1(LbISO_ValueStEntry_flg), ISOValueMeas/Enable  "LbISO_ValueStEntry_flg"
  Initial/1(LbISO_InitiaStMosCmd_flg) -> HVIsoMeasState/1(LbISO_InitiaStMosCmd_flg)
  Initial/2(LbISO_Init2Offline_flg) -> HVIsoMeasState/2(LbISO_Init2Offline_flg)
  Offline/1(LbISO_Offline2PosMeas_flg) -> HVIsoMeasState/3(LbISO_Offline2PosMeas_flg)
  PosMeas/1(LbISO_PosMeas2NegMeas_flg) -> HVIsoMeasState/4(LbISO_PosMeas2NegMeas_flg)
  PosMeas/2(LbISO_PosMeas2Offline_flg) -> HVIsoMeasState/5(LbISO_PosMeas2Offline_flg)
  NegMeas/2(LbISO_NegMeas2VauleCalcu_flg) -> HVIsoMeasState/6(LbISO_NegMeas2VauleCalcu_flg)
  NegMeas/3(LbISO_NegMeas2Offline_flg) -> HVIsoMeasState/7(LbISO_NegMeas2Offline_flg)
  Bus Selector7/1 -> PosMeas/1(LbISO_IsoForbid_flg)  "<LbISO_IsoForbid_flg>"
  Bus Selector7/2 -> PosMeas/2(GcHDP_IsoNegVolt_V)  "<GcHDP_IsoNegVolt_V>"
  Bus Selector7/3 -> PosMeas/3(GcHDP_PackVolt_V)  "<GcHDP_PackVolt_V>"
  Bus Selector8/2 -> NegMeas/2(GcHDP_IsoNegVolt_V)  "<GcHDP_IsoNegVolt_V>"
  Bus Selector8/1 -> NegMeas/1(LbISO_IsoForbid_flg)  "<LbISO_IsoForbid_flg>"
  Bus Selector8/3 -> NegMeas/3(GcHDP_PackVolt_V)  "<GcHDP_PackVolt_V>"
  GbNDP_ReadHVIsoValueVld_flg/1 -> HVIsoValue/3(GbNDP_ReadHVIsoValueVld_flg)
  ISO_GbISO_PosMosCmd_flg/1 -> GbISO_PosMosCmd_flg/1  "GbISO_PosMosCmd_flg"
  ISO_GbISO_NegMosCmd_flg/1 -> GbISO_NegMosCmd_flg/1  "GbISO_NegMosCmd_flg"
  ISOValueMeas/2(GbISO_ResCalFlt_flg) -> GbISO_ResCalFlt_flg/1
  Initial/3(LbISO_InitNegVoltCheck_flg) -> ISO_GbISO_ResInitFlt_flg/1
  ISO_GbISO_ResInitFlt_flg/1 -> GbISO_ResInitFlt_flg/1  "GbISO_ResInitFlt_flg"

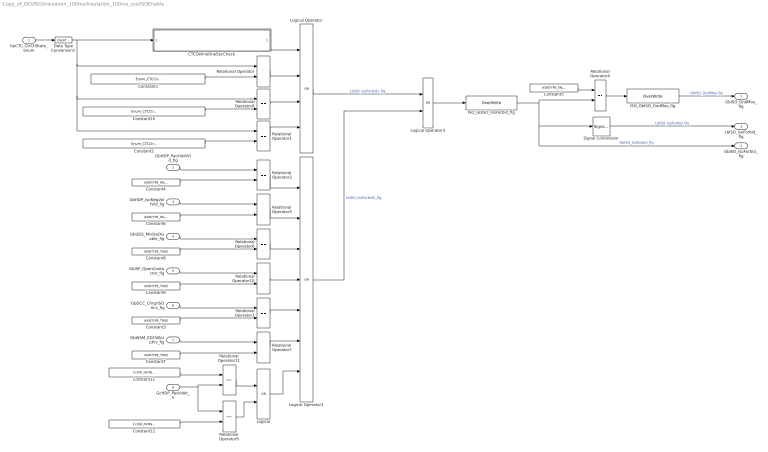
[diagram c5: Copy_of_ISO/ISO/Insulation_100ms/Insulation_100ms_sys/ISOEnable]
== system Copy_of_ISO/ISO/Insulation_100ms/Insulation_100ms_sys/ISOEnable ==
  GeCTC_CtrCtlState_enum : Inport
  GbHDP_PackVoltVld_flg : Inport  Port=2
  GbHDP_IsoNegVoltVld_flg : Inport  Port=3
  GbUDS_MnlIsoDisable_flg : Inport  Port=4
  GbISP_OpenContactor_flg : Inport  Port=5
  GbDCC_ChrgrISOAcv_flg : Inport  Port=6
  GbWSM_EDCWkUpPrs_flg : Inport  Port=7
  GcHDP_PackVolt_V : Inport  Port=8
  CTCOnlineOneSecCheck : Subsystem
  Constant1 : Constant  Value=Enum_CTCCtrCtlState.Enum_CTCCtrCtlState_Connect
  Constant10 : Constant  Value=Enum_CTCCtrCtlState.Enum_CTCCtrCtlState_PreShutdown
  Constant11 : Constant  Value=CcISO_ISOPackVoltMax_V
  Constant12 : Constant  Value=CcISO_ISOPackVoltMin_V
  Constant2 : Constant  Value=Enum_CTCCtrCtlState.Enum_CTCCtrCtlState_Shutdown
  Constant{3,7..9} (4 alike) : Constant  Value=ASWTYPE_TRUE
  Constant4 : Constant  Value=ASWTYPE_FALSE
  Constant5 : Constant  Value=ASWTYPE_FALSE
  Constant6 : Constant  Value=ASWTYPE_FALSE
  Data Type Conversion1 : DataTypeConversion
  ISO_GbISO_GndMos_flg : AIWAYS_Powertrain_BMS_lib/Signals/OverWrite  OverWrite_Value=CbISO_GndMosOvr_flg  OverWrite_flag=CbISO_GndMosOvrSwt_flg
  ISO_GbISO_IsoForbid_flg : AIWAYS_Powertrain_BMS_lib/Signals/OverWrite  OverWrite_Value=CbISO_IsoForbidOvr_flg  OverWrite_flag=CbISO_IsoForbidOvrSwt_flg
  Logical : Logic  Operator=OR  OutDataTypeStr=boolean
  Logical Operator : Logic  Operator=OR  Inputs=4  AllPortsSameDT=off  OutDataTypeStr=boolean
  Logical Operator1 : Logic  Operator=OR  Inputs=7  AllPortsSameDT=off  OutDataTypeStr=boolean
  Logical Operator3 : Logic  Operator=OR  AllPortsSameDT=off  OutDataTypeStr=boolean
  Relational Operator{,1..8,10} (10 alike) : RelationalOperator  Operator===  OutDataTypeStr=boolean
  Relational Operator11 : RelationalOperator  Operator=<=  OutDataTypeStr=boolean
  Relational Operator9 : RelationalOperator  Operator=<=  OutDataTypeStr=boolean
  Signal Conversion : SignalConversion  ConversionOutput=Contiguous copy  OverrideOpt=off
  GbISO_GndMos_flg : Outport
  GbISO_IsoForbid_flg : Outport  Port=2
  LbISO_IsoForbid_flg : Outport  Port=3
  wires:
  Constant1/1 -> Relational Operator/2
  Constant2/1 -> Relational Operator1/2
  GbHDP_PackVoltVld_flg/1 -> Relational Operator2/1
  Constant4/1 -> Relational Operator2/2
  GbHDP_IsoNegVoltVld_flg/1 -> Relational Operator5/1
  Constant6/1 -> Relational Operator5/2
  Logical Operator/1 -> Logical Operator3/1  "LbISO_IsoForbid1_flg"
  Logical Operator1/1 -> Logical Operator3/2  "LbISO_IsoForbid2_flg"
  GeCTC_CtrCtlState_enum/1 -> Data Type Conversion1/1
  GbUDS_MnlIsoDisable_flg/1 -> Relational Operator6/1
  Constant8/1 -> Relational Operator6/2
  Data Type Conversion1/1 -> CTCOnlineOneSecCheck/1(GeCTC_CtrCtlState_enum), Relational Operator/1, Relational Operator8/1, Relational Operator1/1
  Logical Operator3/1 -> ISO_GbISO_IsoForbid_flg/1
  Constant9/1 -> Relational Operator10/2
  GbISP_OpenContactor_flg/1 -> Relational Operator10/1
  CTCOnlineOneSecCheck/1(LbISO_CTCOnlineTimeReach_flg) -> Logical Operator/1
  Relational Operator/1 -> Logical Operator/2
  Relational Operator1/1 -> Logical Operator/4
  Constant3/1 -> Relational Operator3/2
  GbDCC_ChrgrISOAcv_flg/1 -> Relational Operator3/1
  Relational Operator2/1 -> Logical Operator1/1
  Relational Operator5/1 -> Logical Operator1/2
  Relational Operator6/1 -> Logical Operator1/3
  Relational Operator10/1 -> Logical Operator1/4
  Relational Operator3/1 -> Logical Operator1/5
  Constant5/1 -> Relational Operator4/1
  Relational Operator4/1 -> ISO_GbISO_GndMos_flg/1
  ISO_GbISO_GndMos_flg/1 -> GbISO_GndMos_flg/1  "GbISO_GndMos_flg"
  Constant7/1 -> Relational Operator7/2
  GbWSM_EDCWkUpPrs_flg/1 -> Relational Operator7/1
  Relational Operator7/1 -> Logical Operator1/6
  ISO_GbISO_IsoForbid_flg/1 -> Signal Conversion/1, GbISO_IsoForbid_flg/1, Relational Operator4/2  "GbISO_IsoForbid_flg"
  Constant10/1 -> Relational Operator8/2
  Relational Operator8/1 -> Logical Operator/3
  Signal Conversion/1 -> LbISO_IsoForbid_flg/1  "LbISO_IsoForbid_flg"
  Constant11/1 -> Relational Operator11/1
  GcHDP_PackVolt_V/1 -> Relational Operator9/1, Relational Operator11/2
  Constant12/1 -> Relational Operator9/2
  Relational Operator11/1 -> Logical/1
  Relational Operator9/1 -> Logical/2
  Logical/1 -> Logical Operator1/7

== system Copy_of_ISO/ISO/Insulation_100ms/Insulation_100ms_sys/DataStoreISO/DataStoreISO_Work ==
  GcISO_HVIsoValue_kohm : Inport
  Enable : EnablePort  StatesWhenEnabling=reset
  Data Store Write : AIWAYS_Powertrain_BMS_lib/Signals/Data Store Write  DSW=EcNVM_HVIsoValue_kohm
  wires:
  GcISO_HVIsoValue_kohm/1 -> Data Store Write/1

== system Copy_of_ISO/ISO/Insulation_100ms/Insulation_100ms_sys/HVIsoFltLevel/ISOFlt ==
  GcISO_HVIsoValue_kohm : Inport
  GeLDP_CC2St_enum : Inport  Port=2
  GeCTC_CtrCtlState_enum : Inport  Port=3
  LcISO_IsoSecondLevelResThrld_kohm : Inport  Port=4
  LcISO_IsoFirstLevelResThrld_kohm : Inport  Port=5
  LcISO_IsoNormalLevelResThrld_kohm : Inport  Port=6
  Bus Creator : BusCreator  Inputs=6
  Bus Creator2 : BusCreator  Inputs=6
  Bus Selector : BusSelector  OutputSignals=GcISO_HVIsoValue_kohm,GeLDP_CC2St_enum,GeCTC_CtrCtlState_enum,LcISO_IsoSecondLevelResThrld_kohm,LcISO_IsoFirstLevelResThrld_kohm,LcISO_IsoNormalLevelResThrld_kohm
  Bus Selector1 : BusSelector  OutputSignals=GcISO_HVIsoValue_kohm,GeCTC_CtrCtlState_enum,LcISO_IsoSecondLevelResThrld_kohm,LcISO_IsoFirstLevelResThrld_kohm,LcISO_IsoNormalLevelResThrld_kohm
  Bus Selector2 : BusSelector  OutputSignals=GcISO_HVIsoValue_kohm,GeLDP_CC2St_enum,LcISO_IsoSecondLevelResThrld_kohm,LcISO_IsoFirstLevelResThrld_kohm,LcISO_IsoNormalLevelResThrld_kohm,GeCTC_CtrCtlState_enum
  Bus Selector3 : BusSelector  OutputSignals=GbISO_IsoResFltLevel2_flg,GbISO_IsoResFltLevel1_flg,GbISO_IsoHVoffResFltLevel2_flg,GbISO_IsoHVoffResFltLevel1_flg,GbISO_IsoDCResFltLevel2_flg,GbISO_IsoDCResFltLevel1_flg
  Bus Selector4 : BusSelector  OutputSignals=GbISO_IsoResFltLevel2_flg,GbISO_IsoResFltLevel1_flg,GbISO_IsoHVoffResFltLevel2_flg,GbISO_IsoHVoffResFltLevel1_flg,GbISO_IsoDCResFltLevel2_flg,GbISO_IsoDCResFltLevel1_flg
  ISODCFlt : Subsystem
  ISOFltLevel : Subsystem
  ISOHVoffFlt : Subsystem
  ISOHVonFlt : Subsystem
  GeISO_ResFltLvl_enum : Outport
  GbISO_IsoResFltLevel1_flg : Outport  Port=2
  GbISO_IsoResFltLevel2_flg : Outport  Port=3
  GbISO_IsoResFltLevel3_flg : Outport  Port=4
  GbISO_IsoDCResFltLevel1_flg : Outport  Port=5
  GbISO_IsoDCResFltLevel2_flg : Outport  Port=6
  GbISO_IsoHVoffResFltLevel2_flg : Outport  Port=7
  GbISO_IsoHVoffResFltLevel1_flg : Outport  Port=8
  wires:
  GcISO_HVIsoValue_kohm/1 -> Bus Creator/1
  GeLDP_CC2St_enum/1 -> Bus Creator/2
  GeCTC_CtrCtlState_enum/1 -> Bus Creator/3
  LcISO_IsoSecondLevelResThrld_kohm/1 -> Bus Creator/4
  LcISO_IsoFirstLevelResThrld_kohm/1 -> Bus Creator/5
  LcISO_IsoNormalLevelResThrld_kohm/1 -> Bus Creator/6
  ISOFltLevel/1(GeISO_ResFltLvl_enum) -> GeISO_ResFltLvl_enum/1
  Bus Selector/1 -> ISOHVonFlt/1(GcISO_HVIsoValue_kohm)  "<GcISO_HVIsoValue_kohm>"
  Bus Selector/2 -> ISOHVonFlt/2(GeLDP_CC2St_enum)  "<GeLDP_CC2St_enum>"
  Bus Selector/3 -> ISOHVonFlt/3(GeCTC_CtrCtlState_enum)  "<GeCTC_CtrCtlState_enum>"
  Bus Selector/4 -> ISOHVonFlt/4(LcISO_IsoSecondLevelResThrld_kohm)  "<LcISO_IsoSecondLevelResThrld_kohm>"
  Bus Selector/5 -> ISOHVonFlt/5(LcISO_IsoFirstLevelResThrld_kohm)  "<LcISO_IsoFirstLevelResThrld_kohm>"
  Bus Selector/6 -> ISOHVonFlt/6(LcISO_IsoNormalLevelResThrld_kohm)  "<LcISO_IsoNormalLevelResThrld_kohm>"
  Bus Selector1/1 -> ISOHVoffFlt/1(GcISO_HVIsoValue_kohm)  "<GcISO_HVIsoValue_kohm>"
  Bus Selector1/2 -> ISOHVoffFlt/2(GeCTC_CtrCtlState_enum)  "<GeCTC_CtrCtlState_enum>"
  Bus Selector1/3 -> ISOHVoffFlt/3(LcISO_IsoSecondLevelResThrld_kohm)  "<LcISO_IsoSecondLevelResThrld_kohm>"
  Bus Selector1/4 -> ISOHVoffFlt/4(LcISO_IsoFirstLevelResThrld_kohm)  "<LcISO_IsoFirstLevelResThrld_kohm>"
  Bus Selector1/5 -> ISOHVoffFlt/5(LcISO_IsoNormalLevelResThrld_kohm)  "<LcISO_IsoNormalLevelResThrld_kohm>"
  Bus Creator/1 -> Bus Selector2/1, Bus Selector1/1, Bus Selector/1
  Bus Selector2/1 -> ISODCFlt/1(GcISO_HVIsoValue_kohm)  "<GcISO_HVIsoValue_kohm>"
  Bus Selector2/3 -> ISODCFlt/3(LcISO_IsoSecondLevelResThrld_kohm)  "<LcISO_IsoSecondLevelResThrld_kohm>"
  Bus Selector2/4 -> ISODCFlt/4(LcISO_IsoFirstLevelResThrld_kohm)  "<LcISO_IsoFirstLevelResThrld_kohm>"
  Bus Selector2/5 -> ISODCFlt/5(LcISO_IsoNormalLevelResThrld_kohm)  "<LcISO_IsoNormalLevelResThrld_kohm>"
  Bus Selector2/2 -> ISODCFlt/2(GeLDP_CC2St_enum)  "<GeLDP_CC2St_enum>"
  ISOHVonFlt/1(GbISO_IsoResFltLevel3_flg) -> GbISO_IsoResFltLevel3_flg/1
  ISOHVonFlt/2(GbISO_IsoResFltLevel2_flg) -> Bus Creator2/1
  ISOHVonFlt/3(GbISO_IsoResFltLevel1_flg) -> Bus Creator2/2
  ISOHVoffFlt/1(GbISO_IsoHVoffResFltLevel2_flg) -> Bus Creator2/3
  ISOHVoffFlt/2(GbISO_IsoHVoffResFltLevel1_flg) -> Bus Creator2/4
  ISODCFlt/1(GbISO_IsoDCResFltLevel2_flg) -> Bus Creator2/5
  ISODCFlt/2(GbISO_IsoDCResFltLevel1_flg) -> Bus Creator2/6
  Bus Creator2/1 -> Bus Selector4/1, Bus Selector3/1
  Bus Selector3/1 -> ISOFltLevel/1(GbISO_IsoResFltLevel2_flg)  "<GbISO_IsoResFltLevel2_flg>"
  Bus Selector3/2 -> ISOFltLevel/2(GbISO_IsoResFltLevel1_flg)  "<GbISO_IsoResFltLevel1_flg>"
  Bus Selector3/3 -> ISOFltLevel/3(GbISO_IsoHVoffResFltLevel2_flg)  "<GbISO_IsoHVoffResFltLevel2_flg>"
  Bus Selector3/4 -> ISOFltLevel/4(GbISO_IsoHVoffResFltLevel1_flg)  "<GbISO_IsoHVoffResFltLevel1_flg>"
  Bus Selector3/5 -> ISOFltLevel/5(GbISO_IsoDCResFltLevel2_flg)  "<GbISO_IsoDCResFltLevel2_flg>"
  Bus Selector3/6 -> ISOFltLevel/6(GbISO_IsoDCResFltLevel1_flg)  "<GbISO_IsoDCResFltLevel1_flg>"
  Bus Selector4/1 -> GbISO_IsoResFltLevel2_flg/1  "<GbISO_IsoResFltLevel2_flg>"
  Bus Selector4/2 -> GbISO_IsoResFltLevel1_flg/1  "<GbISO_IsoResFltLevel1_flg>"
  Bus Selector4/3 -> GbISO_IsoHVoffResFltLevel2_flg/1  "<GbISO_IsoHVoffResFltLevel2_flg>"
  Bus Selector4/4 -> GbISO_IsoHVoffResFltLevel1_flg/1  "<GbISO_IsoHVoffResFltLevel1_flg>"
  Bus Selector4/5 -> GbISO_IsoDCResFltLevel2_flg/1  "<GbISO_IsoDCResFltLevel2_flg>"
  Bus Selector4/6 -> GbISO_IsoDCResFltLevel1_flg/1  "<GbISO_IsoDCResFltLevel1_flg>"
  Bus Selector2/6 -> ISODCFlt/6(GeCTC_CtrCtlState_enum)  "<GeCTC_CtrCtlState_enum>"

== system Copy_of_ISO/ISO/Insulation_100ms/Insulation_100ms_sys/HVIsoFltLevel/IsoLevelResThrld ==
  GeCTC_CtrCtlState_enum : Inport
  GeCTC_CtrCtlConnMode_enum : Inport  Port=2
  Constant10 : Constant  Value=Enum_CTCCtrCtlConnMode.Enum_CTCCtrCtlConnMode_EDCChrg
  Constant19 : Constant  Value=CcISO_FirLvlResChrg_kohm
  Constant2 : Constant  Value=CcISO_SedLvlResChrg_kohm
  Constant3 : Constant  Value=CcISO_FirLvlResNotChrg_kohm
  Constant4 : Constant  Value=CcISO_SedLvlResNotChrg_kohm
  Constant5 : Constant  Value=CcISO_NorLvlResNotChrg_kohm
  Constant6 : Constant  Value=Enum_CTCCtrCtlConnMode.Enum_CTCCtrCtlConnMode_DCChrg
  Constant7 : Constant  Value=CcISO_NorLvlResChrg_kohm
  Constant8 : Constant  Value=Enum_CTCCtrCtlState.Enum_CTCCtrCtlState_Online
  Constant9 : Constant  Value=Enum_CTCCtrCtlConnMode.Enum_CTCCtrCtlConnMode_ACChrg
  Data Type Conversion1 : DataTypeConversion
  Data Type Conversion2 : DataTypeConversion
  Demux : Demux  Outputs=3
  Logical Operator2 : Logic  Operator=OR  Inputs=3  AllPortsSameDT=off  OutDataTypeStr=boolean
  Logical Operator4 : Logic  AllPortsSameDT=off  OutDataTypeStr=boolean
  Mux : Mux  Inputs=3
  Mux1 : Mux  Inputs=3
  Relational Operator{1..4} (4 alike) : RelationalOperator  Operator===  OutDataTypeStr=boolean
  Signal Conversion1 : SignalConversion  OverrideOpt=off
  Signal Conversion2 : SignalConversion  OverrideOpt=off
  Signal Conversion3 : SignalConversion  OverrideOpt=off
  Switch1 : Switch  Criteria=u2 ~= 0
  LcISO_IsoSecondLevelResThrld_kohm : Outport
  LcISO_IsoFirstLevelResThrld_kohm : Outport  Port=2
  LcISO_IsoNormalLevelResThrld_kohm : Outport  Port=3
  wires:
  Switch1/1 -> Demux/1
  Mux/1 -> Switch1/1
  Mux1/1 -> Switch1/3
  GeCTC_CtrCtlState_enum/1 -> Data Type Conversion1/1
  Constant2/1 -> Mux/1
  Constant19/1 -> Mux/2
  Constant7/1 -> Mux/3
  Signal Conversion1/1 -> LcISO_IsoSecondLevelResThrld_kohm/1  "LcISO_IsoSecondLevelResThrld_kohm"
  Signal Conversion2/1 -> LcISO_IsoFirstLevelResThrld_kohm/1  "LcISO_IsoFirstLevelResThrld_kohm"
  Signal Conversion3/1 -> LcISO_IsoNormalLevelResThrld_kohm/1  "LcISO_IsoNormalLevelResThrld_kohm"
  GeCTC_CtrCtlConnMode_enum/1 -> Data Type Conversion2/1
  Constant6/1 -> Relational Operator2/2
  Constant8/1 -> Relational Operator1/2
  Data Type Conversion1/1 -> Relational Operator1/1
  Constant9/1 -> Relational Operator3/2
  Data Type Conversion2/1 -> Relational Operator2/1, Relational Operator3/1, Relational Operator4/1
  Constant10/1 -> Relational Operator4/2
  Relational Operator2/1 -> Logical Operator2/1
  Relational Operator3/1 -> Logical Operator2/2
  Relational Operator4/1 -> Logical Operator2/3
  Logical Operator2/1 -> Logical Operator4/2
  Relational Operator1/1 -> Logical Operator4/1
  Logical Operator4/1 -> Switch1/2
  Demux/1 -> Signal Conversion1/1
  Demux/2 -> Signal Conversion2/1
  Demux/3 -> Signal Conversion3/1
  Constant4/1 -> Mux1/1
  Constant3/1 -> Mux1/2
  Constant5/1 -> Mux1/3

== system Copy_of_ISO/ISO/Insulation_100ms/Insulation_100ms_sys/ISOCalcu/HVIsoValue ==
  LbISO_ValueStEntry_flg : Inport
  LcISO_HVIsoValue_kohm : Inport  Port=2
  GbNDP_ReadHVIsoValueVld_flg : Inport  Port=3
  Comparison4 : RelationalOperator  Operator===  OutDataTypeStr=boolean
  Constant1 : Constant  Value=CcISO_IsoDefaultValue_kohm
  Constant2 : Constant  Value=ASWTYPE_FALSE
  Constant3 : Constant  Value=CcISO_ISOResNvmMin_kohm
  Constant4 : Constant  Value=ISO_CONST0_NUMB
  Data Store Read : AIWAYS_Powertrain_BMS_lib/Signals/Data Store Read  Priority=0  DSR=EcNVM_HVIsoValue_kohm
  EdgeFalling : AIWAYS_Powertrain_BMS_lib/Logical Operators/EdgeFalling
  ISOValueFilter : Subsystem
  ISO_GcISO_HVIsoValue_kohm : AIWAYS_Powertrain_BMS_lib/Signals/OverWrite  OverWrite_Value=CcISO_HVIsoValueOvr_kohm  OverWrite_flag=CbISO_HVIsoValueOvrSwt_flg
  Logical1 : Logic  Operator=OR  OutDataTypeStr=boolean
  MinMax1 : MinMax  Function=max  Inputs=2  OutDataTypeStr=Inherit: Inherit via back propagation  RndMeth=Zero
  MinMax2 : MinMax  Function=max  Inputs=2  OutDataTypeStr=Inherit: Inherit via back propagation  RndMeth=Zero
  Switch1 : Switch  Criteria=u2 ~= 0
  Switch3 : Switch  Criteria=u2 ~= 0
  Unit Delay1 : UnitDelay  SampleTime=-1  StateName=StateName
  Unit Delay21 : UnitDelay  InitialCondition=ASWTYPE_TRUE  SampleTime=-1  StateName=StateName
  GcISO_HVIsoValue_kohm : Outport
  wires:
  Switch3/1 -> ISO_GcISO_HVIsoValue_kohm/1
  ISO_GcISO_HVIsoValue_kohm/1 -> GcISO_HVIsoValue_kohm/1  "GcISO_HVIsoValue_kohm"
  GbNDP_ReadHVIsoValueVld_flg/1 -> Switch1/2
  Data Store Read/1 -> MinMax1/2
  Constant1/1 -> Switch1/3
  Unit Delay21/1 -> Logical1/1
  Switch1/1 -> Switch3/1  "LcISO_HVIsoNvmValue_kohm"
  Constant2/1 -> Unit Delay21/1
  LbISO_ValueStEntry_flg/1 -> EdgeFalling/1
  LcISO_HVIsoValue_kohm/1 -> ISOValueFilter/1(LcISO_HVIsoValue_kohm)
  EdgeFalling/1 -> ISOValueFilter/Enable
  MinMax1/1 -> Switch1/1
  Constant3/1 -> MinMax1/1
  ISOValueFilter/1(LcISO_HVIsoValueFilter_kohm) -> Switch3/3, MinMax2/2
  Constant4/1 -> Comparison4/1
  Logical1/1 -> Switch3/2  "LbISO_HVIsoNvmCalcSw_flg"
  Comparison4/1 -> Logical1/2
  MinMax2/1 -> Unit Delay1/1, Comparison4/2
  Unit Delay1/1 -> MinMax2/1

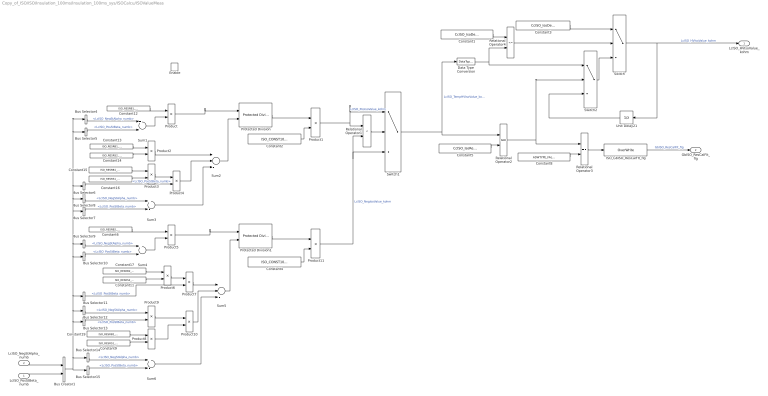
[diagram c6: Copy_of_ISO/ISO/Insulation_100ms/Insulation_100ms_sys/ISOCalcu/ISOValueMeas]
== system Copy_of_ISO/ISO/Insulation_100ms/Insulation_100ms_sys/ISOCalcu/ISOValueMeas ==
  LcISO_PosStBeta_numb : Inport
  LcISO_NegStAlpha_numb : Inport  Port=2
  Enable : EnablePort
  Bus Creator1 : BusCreator  Inputs=2
  Bus Selector{5..7,10..11,13,15} (7 alike) : BusSelector  OutputSignals=LcISO_PosStBeta_numb
  Bus Selector{4,8..9,12,14} (5 alike) : BusSelector  OutputSignals=LcISO_NegStAlpha_numb
  Constant1 : Constant  Value=CcISO_IsoDefaultValue_kohm
  Constant11 : Constant  Value=ISO_RESRS2_OHM
  Constant12 : Constant  Value=ISO_RESRB1_OHM
  Constant13 : Constant  Value=ISO_RESRB1_OHM
  Constant14 : Constant  Value=ISO_RESRS2_OHM
  Constant15 : Constant  Value=ISO_RESRB1_OHM
  Constant16 : Constant  Value=ISO_RESRS1_OHM
  Constant17 : Constant  Value=ISO_RESRB2_OHM
  Constant19 : Constant  Value=ISO_RESRB2_OHM
  Constant2 : Constant  Value=ISO_CONST1000_NUMB
  Constant3 : Constant  Value=CcISO_IsoDefaultValue_kohm
  Constant4 : Constant  Value=ISO_CONST1000_NUMB
  Constant5 : Constant  Value=CcISO_IsoResVldVal_NUMB
  Constant6 : Constant  Value=ISO_RESRB2_OHM
  Constant8 : Constant  Value=ASWTYPE_FALSE
  Constant9 : Constant  Value=ISO_RESRS1_OHM
  Data Type Conversion : DataTypeConversion
  ISO_GbISO_ResCalFlt_flg : AIWAYS_Powertrain_BMS_lib/Signals/OverWrite  OverWrite_Value=CbISO_ResCalFltOvr_flg  OverWrite_flag=CbISO_ResCalFltOvrSwt_flg
  Product{,4..5,7,9..10} (6 alike) : Product  OutDataTypeStr=Inherit: Inherit via back propagation
  Product{1..3,6,8,11} (6 alike) : Product  Inputs=*/  OutDataTypeStr=Inherit: Inherit via back propagation
  Protected Division : AIWAYS_Powertrain_BMS_lib/Arithmetic Operators/Protected Division
  Protected Division1 : AIWAYS_Powertrain_BMS_lib/Arithmetic Operators/Protected Division
  Relational Operator1 : RelationalOperator  Operator=<  OutDataTypeStr=boolean
  Relational Operator2 : RelationalOperator  OutDataTypeStr=boolean
  Relational Operator3 : RelationalOperator  Operator===  OutDataTypeStr=boolean
  Relational Operator4 : RelationalOperator  Operator=<=  OutDataTypeStr=boolean
  Sum{1,3..4,6} (4 alike) : Sum  Inputs=+-  OutDataTypeStr=Inherit: Inherit via back propagation  RndMeth=Zero
  Sum2 : Sum  Inputs=++-  OutDataTypeStr=Inherit: Inherit via back propagation  RndMeth=Zero
  Sum5 : Sum  Inputs=++-  OutDataTypeStr=Inherit: Inherit via back propagation  RndMeth=Zero
  Switch : Switch  Criteria=u2 ~= 0
  Switch1 : Switch  Criteria=u2 ~= 0  Threshold=1  RndMeth=Zero
  Switch2 : Switch  Criteria=u2 ~= 0
  Unit Delay21 : UnitDelay  SampleTime=-1  StateName=StateName
  LcISO_HVIsoValue_kohm : Outport
  GbISO_ResCalFlt_flg : Outport  Port=2
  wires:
  Relational Operator4/1 -> Switch/2
  Constant3/1 -> Switch/1
  Switch1/1 -> Data Type Conversion/1, Relational Operator2/1  "LcISO_TempHVIsoValue_kohm"
  Constant1/1 -> Relational Operator4/1
  LcISO_NegStAlpha_numb/1 -> Bus Creator1/1
  LcISO_PosStBeta_numb/1 -> Bus Creator1/2
  Sum1/1 -> Product/2
  Constant12/1 -> Product/1
  Constant13/1 -> Product2/1
  Constant14/1 -> Product2/2
  Constant15/1 -> Product3/1
  Constant16/1 -> Product3/2
  Product3/1 -> Product4/1
  Bus Selector6/1 -> Product4/2  "<LcISO_PosStBeta_numb>"
  Sum3/1 -> Sum2/3
  Product2/1 -> Sum2/1
  Product4/1 -> Sum2/2
  Bus Selector12/1 -> Product9/1  "<LcISO_NegStAlpha_numb>"
  Bus Selector13/1 -> Product9/2  "<LcISO_PosStBeta_numb>"
  Bus Selector11/1 -> Product7/2  "<LcISO_PosStBeta_numb>"
  Constant6/1 -> Product5/1
  Sum4/1 -> Product5/2
  Constant17/1 -> Product6/1
  Constant11/1 -> Product6/2
  Product6/1 -> Product7/1
  Product8/1 -> Product10/2
  Constant9/1 -> Product8/2
  Constant19/1 -> Product8/1
  Product9/1 -> Product10/1
  Product7/1 -> Sum5/1
  Product10/1 -> Sum5/2
  Sum6/1 -> Sum5/3
  Bus Creator1/1 -> Bus Selector4/1, Bus Selector5/1, Bus Selector6/1, Bus Selector8/1, Bus Selector7/1, Bus Selector9/1, Bus Selector10/1, Bus Selector11/1, Bus Selector12/1, Bus Selector13/1, Bus Selector14/1, Bus Selector15/1
  Relational Operator1/1 -> Switch1/2
  Constant2/1 -> Product1/2
  Constant4/1 -> Product11/2
  Switch2/1 -> Switch/3
  Relational Operator2/1 -> Relational Operator3/1, Switch2/2
  Constant5/1 -> Relational Operator2/2
  Constant8/1 -> Relational Operator3/2
  Relational Operator3/1 -> ISO_GbISO_ResCalFlt_flg/1
  ISO_GbISO_ResCalFlt_flg/1 -> GbISO_ResCalFlt_flg/1  "GbISO_ResCalFlt_flg"
  Product1/1 -> Switch1/1, Relational Operator1/1  "LcISO_PosIsoValue_kohm"
  Product11/1 -> Relational Operator1/2, Switch1/3  "LcISO_NegIsoValue_kohm"
  Switch/1 -> Unit Delay21/1, LcISO_HVIsoValue_kohm/1  "LcISO_HVIsoValue_kohm"
  Bus Selector5/1 -> Sum1/2  "<LcISO_PosStBeta_numb>"
  Bus Selector4/1 -> Sum1/1  "<LcISO_NegStAlpha_numb>"
  Bus Selector8/1 -> Sum3/1  "<LcISO_NegStAlpha_numb>"
  Bus Selector7/1 -> Sum3/2  "<LcISO_PosStBeta_numb>"
  Bus Selector9/1 -> Sum4/1  "<LcISO_NegStAlpha_numb>"
  Bus Selector10/1 -> Sum4/2  "<LcISO_PosStBeta_numb>"
  Bus Selector14/1 -> Sum6/1  "<LcISO_NegStAlpha_numb>"
  Bus Selector15/1 -> Sum6/2  "<LcISO_PosStBeta_numb>"
  Product/1 -> Protected Division/1
  Protected Division/1 -> Product1/1
  Sum2/1 -> Protected Division/2
  Protected Division1/1 -> Product11/1
  Product5/1 -> Protected Division1/1
  Sum5/1 -> Protected Division1/2
  Unit Delay21/1 -> Switch2/3
  Data Type Conversion/1 -> Switch2/1, Relational Operator4/2
